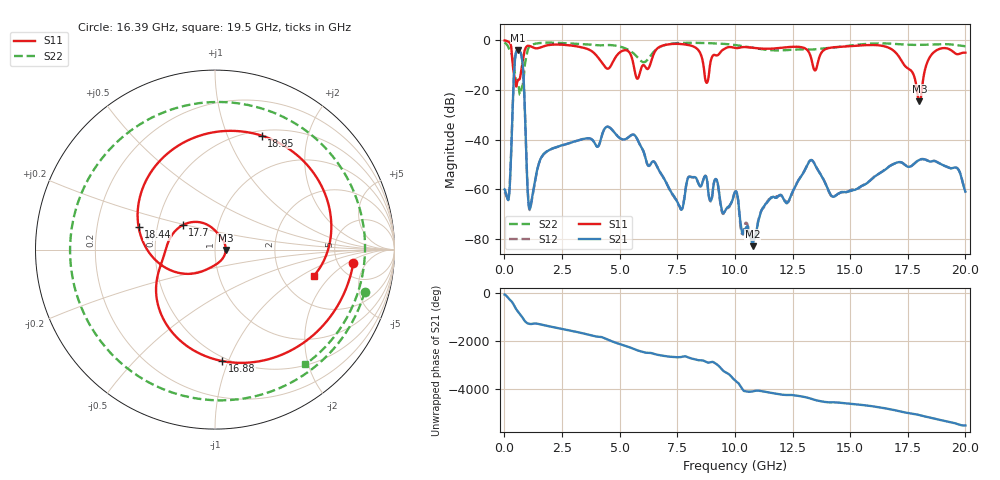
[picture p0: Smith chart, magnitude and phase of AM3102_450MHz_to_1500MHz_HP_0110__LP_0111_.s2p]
!Agilent Technologies,E8364B,MY43040894,A.07.50.67
!Agilent E8364B: A.07.50.67
!Date: Thursday, January 11, 2018 05:47:30
!Correction: S11(Full 2 Port(1,2))
!S21(Full 2 Port(1,2))
!S12(Full 2 Port(1,2))
!S22(Full 2 Port(1,2))
!S2P File: Measurements: S11, S21, S12, S22:
# Hz S  dB  R 50
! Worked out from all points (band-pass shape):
!   1601 points, 10 MHz to 20 GHz, reference 50 ohm
!   highest |S21| = -3.92 dB at 597.2 MHz (marker M1); lowest = -82.8 dB at 10.78 GHz (marker M2)
!   |S21| within 3 dB of the highest: 469.5 MHz to 756.2 MHz (286.7 MHz wide, 46.8 % of centre)
!   lowest |S11| = -24.5 dB at 18 GHz (marker M3), VSWR 1.13, Z = 56.3 - j0.306 ohm
!   |S11| at or under -10 dB: 364.6 MHz to 766.7 MHz (402.2 MHz wide, 71.1 % of centre); 5.606 GHz to 6.02 GHz (413.6 MHz wide, 7.11 % of centre); 17.35 GHz to 18.3 GHz (951.2 MHz wide, 5.34 % of centre)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
!   |S22| runs from -21.9 to -0.8 dB; largest |S21 - S12| = 0.0021
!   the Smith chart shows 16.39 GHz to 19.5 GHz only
!   S11 on the Smith chart (normalised r, x): 16.39 GHz: 6.91, -2.54; 16.88 GHz: 0.47, -0.95; 17.7 GHz: 0.67, +0.19; 18.44 GHz: 0.39, +0.12; 18.95 GHz: 0.56, +1.33; 19.5 GHz: 3.03, -1.31
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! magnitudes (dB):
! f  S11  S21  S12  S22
! 10 MHz  -0.1  -60.0  -61.1  -0.8
! 197.4 MHz  -0.7  -63.0  -62.4  -3.3
! 597.2 MHz  -15.9  -3.9  -3.9  -18.2
! 784.6 MHz  -9.1  -8.9  -8.9  -18.2
! 1.109 GHz  -2.3  -67.8  -68.2  -2.4
! 1.697 GHz  -2.4  -45.9  -45.9  -1.0
! 3.346 GHz  -2.8  -39.9  -39.9  -1.5
! 6.682 GHz  -2.9  -51.9  -51.9  -3.1
! 8.781 GHz  -17.1  -55.8  -55.8  -1.1
! 10.01 GHz  -3.1  -61.0  -61.0  -1.9
! 10.78 GHz  -3.0  -82.8  -79.2  -3.0
! 13.34 GHz  -8.4  -48.3  -48.3  -3.7
! 14.25 GHz  -2.9  -62.9  -63.1  -3.0
! 16.39 GHz  -2.2  -52.9  -52.8  -1.2
! 16.68 GHz  -3.0  -50.9  -50.8  -1.3
! 16.88 GHz  -4.1  -49.8  -49.8  -1.4
! 17.7 GHz  -12.9  -50.3  -50.3  -1.8
! 18 GHz  -24.5  -48.1  -48.1  -1.9
! 18.44 GHz  -7.1  -48.8  -48.7  -1.7
! 18.95 GHz  -3.3  -49.9  -49.9  -1.5
! 19.5 GHz  -4.9  -51.3  -51.3  -1.8
! 20 GHz  -5.0  -60.9  -60.1  -2.4
